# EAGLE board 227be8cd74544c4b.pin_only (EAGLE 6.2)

Size 13.97 x 21.59 mm. Coordinates in mm from the lower left corner, seen from the top.
Outline: 0,19.05 0,2.54 arc90 2.54,0 11.43,0 arc90 13.97,2.54 13.97,19.05 arc90 11.43,21.59 2.54,21.59 arc90 0,19.05
Copper layers (1*16): Top 0.035mm / dielectric 1.5mm / Bottom 0.035mm
Design rules: minimum track width 8mil, minimum drill 0.4mm, track to track 8mil, track to pad 8mil, pad to pad 8mil, via to via 8mil, smd to smd 8mil, copper to edge 20mil, drill to drill 8mil, minimum pad ring 8mil, minimum via ring 10mil, stop-mask expansion 3mil, vias tented up to drill 20mil, thermal gap 8mil

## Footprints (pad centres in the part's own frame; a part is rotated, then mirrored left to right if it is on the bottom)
0805 = smd 1.3 x 1.5: 1 -0.95,0; 2 0.95,0
FIDUCIAL_1MM = smd 1 x 1: 1 0,0
1X03_ROUND_76 = drill 1 pad 1.93: 1 -2.54,0; 2 0,0; 3 2.54,0
ELECTRET_9.7 = drill 0.6 pad 1.778: + 1.3,2; - -1.3,2
SC70-5 = smd 0.35 x 1.15: 1 -0.65,-0.85; 2 0,-0.85; 3 0.65,-0.85; 4 0.65,0.85; 5 -0.65,0.85
MOUNTINGHOLE_2.5_PLATED = drill 2.5 pad 3.2: P$1 0,0
TRIMPOT_BOURNS_TC33X-2 = smd 1.2 x 1.2: 1 -1,-1.8; 3 1,-1.8 | smd 1.6 x 1.5: 2 0,1.45

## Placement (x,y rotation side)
C1  0.1µF  [0805]  7.11,11.43 180 top
C2  0.01uF  [0805]  2.54,13.97 180 top
C3  100pF  [0805]  12.57,5.71 90 top
C4  10uF  [0805]  11.56,11.05 180 top
FB1  FERRITE  [0805]  3.56,5.71 90 top
FB2  FERRITE  [0805]  1.52,5.71 270 top
FID1  FIDUCIAL""  [FIDUCIAL_1MM]  12.45,2.41 0 top
FID2  FIDUCIAL""  [FIDUCIAL_1MM]  1.65,16.26 0 top
JP1  [1X03_ROUND_76]  7.11,1.52 0 top
Q1  CMA-4544PF-W  [ELECTRET_9.7]  6.99,14.1 0 bottom
R1  1K  [0805]  7.11,13.72 0 top
R2  1K  [0805]  10.67,14.1 270 top
R3  1M  [0805]  3.56,10.67 90 top
R4  1M  [0805]  1.52,10.67 270 top
R5  1K  [0805]  11.56,8.89 180 top
R7  22K  [0805]  5.59,5.71 270 top
U1  MAX4466EXK+T  [SC70-5]  7.62,8.89 270 top
U$11  MOUNTINGHOLE2.5  [MOUNTINGHOLE_2.5_PLATED]  2.16,19.3 0 top
U$14  MOUNTINGHOLE2.5  [MOUNTINGHOLE_2.5_PLATED]  11.81,19.3 0 top
U$16  [ADAFRUIT_2.5MM]  5.33,18.16 0 top
U$17  [ADAFRUIT_2.5MM]  8.13,19.05 0 bottom
VR1  TC33X-2-104E (100K)  [TRIMPOT_BOURNS_TC33X-2]  9.27,5.46 270 top

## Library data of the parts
C1-C4 FB1 FB2 FID1 FID2 JP1 Q1 R1-R5 R7 U1 U$11 U$14 U$16 U$17 VR1 = microbuilder

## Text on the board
tPlace: MAX4466 | MIC AMP | VCC | GND | OUT
bPlace: VCC: 2.4-5.5V | Adjustable gain | VCC | GND | OUT

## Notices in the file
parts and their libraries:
microbuilder: This work is placed in the public domain, and may be freely used for commercial and non-commercial work with the following conditions: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
